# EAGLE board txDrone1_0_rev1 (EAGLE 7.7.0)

Size 100 x 80 mm. Coordinates in mm from the lower left corner, seen from the top.
Outline: 0,0 100,0 100,80 0,80 0,0
Copper layers (1*16): Top 0.035mm / dielectric 1.5mm / Bottom 0.035mm
Design rules "default *": minimum track width 10mil, minimum drill 24mil, track to track 8mil, track to pad 8mil, pad to pad 8mil, via to via 8mil, smd to smd 8mil, copper to edge 40mil, drill to drill 8mil, minimum pad ring 10mil, minimum via ring 8mil, stop-mask expansion 16mil, vias tented up to drill 0mil, thermal gap 10mil

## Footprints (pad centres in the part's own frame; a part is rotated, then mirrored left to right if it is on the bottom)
0805-CAP = smd 0.8 x 1.2: 1 -0.9,0; 2 0.9,0
SCREWTERMINAL-3.5MM-6@1 = drill 1.2 pad 2.032 square: 1 0,0 | drill 1.2 pad 2.032: 2 3.5,0; 3 7,0; 4 10.5,0; 5 14,0; 6 17.5,0
LED-1206 = smd 1.2 x 1.4: A -1.5,0; C 1.5,0
0805 = smd 0.8 x 1.2: 1 -0.9,0; 2 0.9,0
SO08 = smd 0.6 x 2.2: 1 -1.905,-2.6; 2 -0.635,-2.6; 3 0.635,-2.6; 4 1.905,-2.6; 5 1.905,2.6; 6 0.635,2.6; 7 -0.635,2.6; 8 -1.905,2.6
BU-SMA-V = drill 1.27: 1 0,0 | drill 1.778: 2 -2.55,2.55; 3 2.55,2.55; 4 2.55,-2.55; 5 -2.55,-2.55
HC49U-V = drill 0.813: 1 -2.413,0; 2 2.413,0

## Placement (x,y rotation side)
CB0  220nF  [0805-CAP]  9.53,15.88 0 top
CB1  330pF  [0805-CAP]  31.11,8.89 180 top
CM1  1.8pF  [0805-CAP]  31.11,15.24 0 top
CM2  5.6pF  [0805-CAP]  34.92,15.24 180 top
CM3  68pF  [0805-CAP]  31.11,18.41 0 top
CX1  27pF  [0805-CAP]  9.53,19.05 180 top
J1  [SCREWTERMINAL-3.5MM-6@1]  3.81,21.59 270 top
LED1  [LED-1206]  26.67,5.08 180 top
LM  12nH  [0805]  34.92,18.41 0 top
LT  15nH  [0805]  31.11,12.06 180 top
R1  220  [0805]  31.11,5.08 0 top
U$1  TH72032NORMAL  [SO08]  22.86,14.61 270 top
X1  BU-SMA-V  [BU-SMA-V]  45.72,15.24 0 top
XTAL  [HC49U-V]  14.61,16.51 270 top

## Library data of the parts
CB0 CB1 CM1-CM3 CX1 = SparkFun-Capacitors; PROD_ID: CAP-11624
J1 = SparkFun-Connectors
LED1 = SparkFun-LED
LM LT = SparkFun-Passives
R1 = SparkFun-Resistors
U$1 = th72032
X1 = con-coax; OC_FARNELL: unknown; OC_NEWARK: unknown
XTAL = SparkFun-FreqCtrl

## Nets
GND: CB0.2 CB1.2 CM1.2 CM2.2 CX1.2 J1.1 J1.6 LED1.C U$1.2 U$1.8 X1.2 X1.3 X1.4 X1.5
N$1: CM1.1 CM3.1 LT.2 U$1.7
N$2: CM3.2 LM.1
N$3: CM2.1 LM.2 X1.1
N$4: U$1.3 XTAL.2
N$5: CX1.1 XTAL.1
N$6: J1.3 U$1.1
N$7: J1.4 U$1.4
N$8: LED1.A R1.1
VCC: CB0.1 CB1.1 J1.2 J1.5 LT.1 R1.2 U$1.5 U$1.6

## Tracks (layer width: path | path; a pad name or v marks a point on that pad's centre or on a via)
GND  (13 unrouted)
N$1  (3 unrouted)
N$2  (1 unrouted)
N$3  (2 unrouted)
N$4  (1 unrouted)
N$5  (1 unrouted)
N$6  (1 unrouted)
N$7  (1 unrouted)
N$8  (1 unrouted)
VCC  (7 unrouted)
